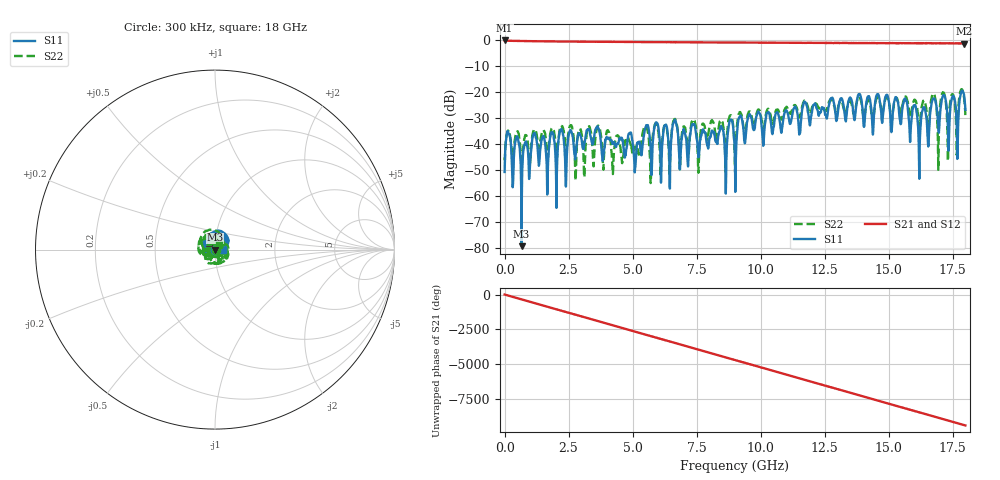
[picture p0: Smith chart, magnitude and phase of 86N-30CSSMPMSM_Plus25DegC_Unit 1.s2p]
!Agilent Technologies,N5230A,MY45000342,A.06.04.32
!Agilent N5230A: A.06.04.32
!Date: Thursday, March 12, 2026 14:21:27
!Correction: S11(Full 2 Port(1,4)) S41(Full 2 Port(1,4)) S14(Full 2 Port(1,4)) S44(Full 2 Port(1,4))
!S2P File: Measurements: S11, S41, S14, S44:
# Hz S  dB  R 50
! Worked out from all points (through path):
!   1601 points, 300 kHz to 18 GHz, reference 50 ohm
!   highest |S21| = 0.01 dB at 300 kHz (marker M1); lowest = -1.2 dB at 17.96 GHz (marker M2)
!   group delay of S21, straight-line fit = 1.46 ns
!   lowest |S11| = -79.2 dB at 664 MHz (marker M3), VSWR 1.00, Z = 50 - j0.00826 ohm
!   |S11| at or under -10 dB: start of sweep to end of sweep
!   |S22| runs from -54.9 to -18.7 dB; largest |S21 - S12| = 0.018
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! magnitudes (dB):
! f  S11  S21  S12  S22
! 300 kHz  -50.6  0.0  0.0  -45.0
! 146.5 MHz  -35.6  -0.1  -0.2  -34.8
! 664 MHz  -79.2  -0.2  -0.3  -48.5
! 1.159 GHz  -35.7  -0.3  -0.3  -34.2
! 1.665 GHz  -59.3  -0.4  -0.4  -43.7
! 1.845 GHz  -35.4  -0.4  -0.4  -33.7
! 2.014 GHz  -54.7  -0.4  -0.4  -42.5
! 3.004 GHz  -37.9  -0.5  -0.5  -35.7
! 6.008 GHz  -33.5  -0.6  -0.7  -35.3
! 8.64 GHz  -58.9  -0.8  -0.8  -48.2
! 8.82 GHz  -30.6  -0.8  -0.8  -28.9
! 9 GHz  -46.2  -0.8  -0.8  -50.5
! 9.203 GHz  -29.1  -0.8  -0.9  -27.6
! 12 GHz  -27.7  -0.9  -1.0  -25.9
! 15.01 GHz  -23.3  -1.0  -1.0  -23.3
! 16.2 GHz  -53.2  -1.1  -1.1  -33.2
! 16.75 GHz  -22.4  -1.1  -1.1  -20.4
! 16.94 GHz  -33.7  -1.1  -1.1  -49.8
! 17.12 GHz  -21.3  -1.1  -1.2  -20.1
! 17.31 GHz  -32.7  -1.1  -1.1  -46.1
! 17.96 GHz  -21.5  -1.2  -1.2  -22.4
! 18 GHz  -26.7  -1.1  -1.2  -28.7
